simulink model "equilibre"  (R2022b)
settings: Solver=VariableStepAuto  StartTime=0.0  StopTime=1.0  RelTol=1e-3

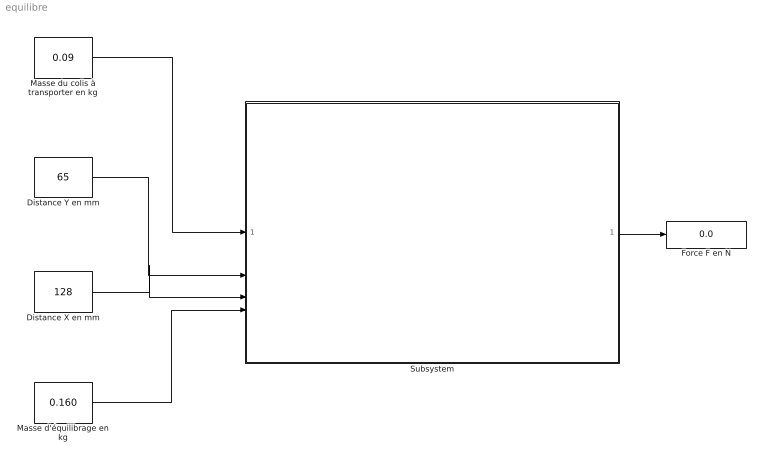
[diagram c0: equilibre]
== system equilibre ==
  Distance X en mm : Constant  Value=128
  Distance Y en mm : Constant  Value=65
  Force F en N : Display
  Masse d'équilibrage en kg : Constant  Value=0.160
  Masse du colis à transporter en kg : Constant  Value=0.09
  Subsystem : Subsystem
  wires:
  Masse du colis à transporter en kg/1 -> Subsystem/1(In1)
  Distance Y en mm/1 -> Subsystem/2(In2)
  Distance X en mm/1 -> Subsystem/3(In3)
  Masse d'équilibrage en kg/1 -> Subsystem/4(In4)
  Subsystem/1(Out2) -> Force F en N/1

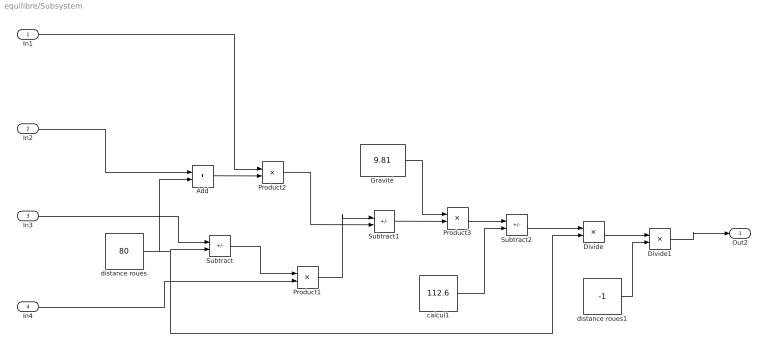
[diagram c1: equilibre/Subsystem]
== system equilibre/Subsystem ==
  In1 : Inport
  In2 : Inport  Port=2
  In3 : Inport  Port=3
  In4 : Inport  Port=4
  Add : Sum
  Divide : Product  Inputs=*/
  Divide1 : Product  Inputs=**
  Gravité : Constant  Value=9.81
  Product1 : Product
  Product2 : Product
  Product3 : Product
  Subtract : Sum  Inputs=+-
  Subtract1 : Sum  Inputs=+-
  Subtract2 : Sum  Inputs=+-
  calcul1 : Constant  Value=112.6
  distance roues : Constant  Value=80
  distance roues1 : Constant  Value=-1
  Out2 : Outport
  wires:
  In3/1 -> Subtract/1
  distance roues/1 -> Add/2, Divide/2, Subtract/2
  In4/1 -> Product1/2
  Subtract/1 -> Product1/1
  In2/1 -> Add/1
  Add/1 -> Product2/2
  In1/1 -> Product2/1
  Product1/1 -> Subtract1/1
  Product2/1 -> Subtract1/2
  Subtract1/1 -> Product3/2
  Gravité/1 -> Product3/1
  Product3/1 -> Subtract2/1
  calcul1/1 -> Subtract2/2
  Subtract2/1 -> Divide/1
  Divide1/1 -> Out2/1
  Divide/1 -> Divide1/1
  distance roues1/1 -> Divide1/2
